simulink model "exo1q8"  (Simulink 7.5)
settings: Solver=ode45  StartTime=0.0  StopTime=10.0  RelTol=1e-3
libraries: fuzblock x1

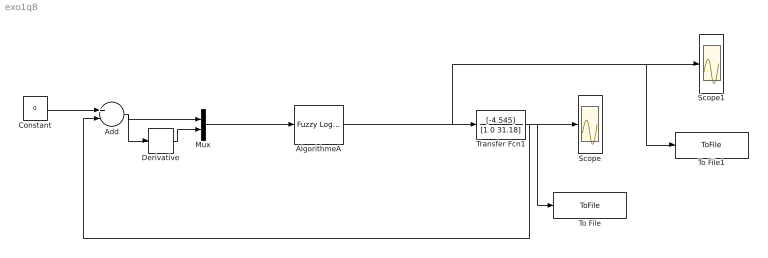
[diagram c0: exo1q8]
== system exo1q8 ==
  Add : Sum  Inputs=+-  OutDataType=fixdt(1, 16)  OutScaling=2^-10
  AlgorithmeA : fuzblock/Fuzzy Logic  Controller  SystemSampleTime=-1  fis=flouA
  Constant : Constant  Value=0  OutDataType=fixdt(1, 16)  OutScaling=2^0
  Derivative : Derivative
  Mux : Mux  Inputs=2
  Scope : Scope
  Scope1 : Scope
  To File : ToFile  Filename=penduleftA.mat
  To File1 : ToFile  Filename=flou
  Transfer Fcn1 : TransferFcn  Numerator=[-4.545]  Denominator=[1 0 31.18]
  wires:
  Transfer Fcn1/1 -> Scope/1, To File/1, Add/2
  Constant/1 -> Add/1
  Add/1 -> Mux/1, Derivative/1
  Derivative/1 -> Mux/2
  Mux/1 -> AlgorithmeA/1
  AlgorithmeA/1 -> Transfer Fcn1/1, Scope1/1, To File1/1
